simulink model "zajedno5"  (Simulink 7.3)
settings: Solver=ode3  StartTime=0.0  StopTime=350  FixedStep=0.1  RelTol=1e-3
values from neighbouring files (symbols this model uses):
  alpha_r = 3.6    [test3.m]
  alpha_u = 27    [test3.m]
  alpha_v = 26    [test3.m]
  beta_r = 0    [test3.m]
  beta_rr = 2.5    [test3.m]
  beta_u = 0    [test3.m]
  beta_uu = 56    [test3.m]
  beta_v = 0    [test3.m]
  beta_vv = 47    [test3.m]
undefined symbols (not defined in the file or in its folder): Charli, Regulatori_Charli
libraries: simulink x2, fuzblock x1

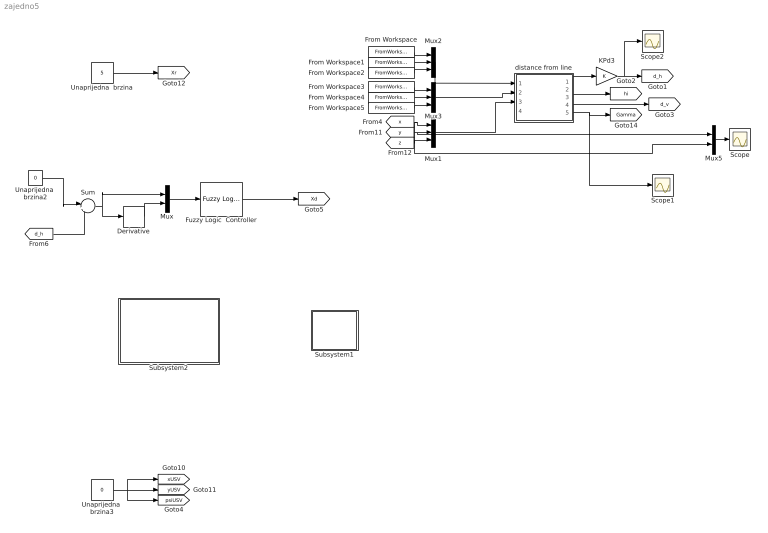
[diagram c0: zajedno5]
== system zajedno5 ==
  Derivative : Derivative
  From Workspace : FromWorkspace  VariableName=[t, n1]  SampleTime=0  Interpolate=off  OutputAfterFinalValue=Holding final value
  From Workspace1 : FromWorkspace  VariableName=[t, e1]  SampleTime=0  Interpolate=off  OutputAfterFinalValue=Holding final value
  From Workspace2 : FromWorkspace  VariableName=[t, d1]  SampleTime=0  Interpolate=off  OutputAfterFinalValue=Holding final value
  From Workspace3 : FromWorkspace  VariableName=[t, n2]  SampleTime=0  Interpolate=off  OutputAfterFinalValue=Holding final value
  From Workspace4 : FromWorkspace  VariableName=[t, e2]  SampleTime=0  Interpolate=off  OutputAfterFinalValue=Holding final value
  From Workspace5 : FromWorkspace  VariableName=[t, d2]  SampleTime=0  Interpolate=off  OutputAfterFinalValue=Holding final value
  Fuzzy Logic  Controller : fuzblock/Fuzzy Logic  Controller  SystemSampleTime=-1  fis=regulator
  KPd3 : Gain  ParameterDataType=sfix(16)  ParameterScaling=2^0  OutDataType=sfix(16)  OutScaling=2^0
  Mux : Mux  Inputs=2
  Mux1 : Mux  Inputs=3
  Mux2 : Mux  Inputs=3
  Mux3 : Mux  Inputs=3
  Mux5 : Mux  Inputs=2
  Scope : Scope
  Scope1 : Scope
  Scope2 : Scope
  Subsystem1 : Subsystem
  Subsystem2 : Subsystem
  Sum : Sum  Inputs=|+-  OutDataType=fixdt(1, 16)  OutScaling=2^0
  Unaprijedna  brzina : Constant  Value=5  OutDataType=sfix(16)  OutScaling=2^0
  Unaprijedna  brzina2 : Constant  Value=0  OutDataType=sfix(16)  OutScaling=2^0
  Unaprijedna  brzina3 : Constant  Value=0  OutDataType=sfix(16)  OutScaling=2^0
  distance from line : Subsystem
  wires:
  Mux1/1 -> distance from line/3(T0)
  [x] -> Mux1/1, Mux5/2
  [y] -> Mux1/2, Mux5/1
  [z] -> Mux1/3
  Mux2/1 -> distance from line/1(T1)
  Mux3/1 -> distance from line/2(T2)
  distance from line/1(d_h) -> KPd3/1
  distance from line/2(hi) -> [hi]
  From Workspace/1 -> Mux2/1
  From Workspace1/1 -> Mux2/2
  From Workspace2/1 -> Mux2/3
  From Workspace3/1 -> Mux3/1
  From Workspace4/1 -> Mux3/2
  From Workspace5/1 -> Mux3/3
  distance from line/4(Gamma) -> [Gamma], Scope1/1
  KPd3/1 -> [d_h], Scope2/1
  distance from line/3(d_v) -> [d_v]
  Unaprijedna  brzina2/1 -> Sum/1
  Unaprijedna  brzina3/1 -> [xUSV], [yUSV], [psiUSV]
  Mux5/1 -> Scope/1
  Sum/1 -> Mux/1, Derivative/1
  Derivative/1 -> Mux/2
  Mux/1 -> Fuzzy Logic  Controller/1
  Unaprijedna  brzina/1 -> [Xr]
  Fuzzy Logic  Controller/1 -> [Xd]
  [d_h] -> Sum/2

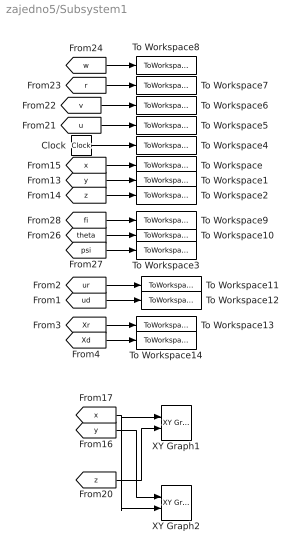
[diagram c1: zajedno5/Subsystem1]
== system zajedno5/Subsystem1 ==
  Clock : Clock
  To Workspace : ToWorkspace  VariableName=x  SampleTime=0.1  SaveFormat=Array
  To Workspace1 : ToWorkspace  VariableName=y  SampleTime=0.1  SaveFormat=Array
  To Workspace10 : ToWorkspace  VariableName=theta  SampleTime=0.1  SaveFormat=Array
  To Workspace11 : ToWorkspace  VariableName=ur  SampleTime=0.1  SaveFormat=Array
  To Workspace12 : ToWorkspace  VariableName=ud  SampleTime=0.1  SaveFormat=Array
  To Workspace13 : ToWorkspace  VariableName=Xr  SampleTime=0.1  SaveFormat=Array
  To Workspace14 : ToWorkspace  VariableName=Xd  SampleTime=0.1  SaveFormat=Array
  To Workspace2 : ToWorkspace  VariableName=z  SampleTime=0.1  SaveFormat=Array
  To Workspace3 : ToWorkspace  VariableName=psi  SampleTime=0.1  SaveFormat=Array
  To Workspace4 : ToWorkspace  VariableName=time  SampleTime=0.1  SaveFormat=Array
  To Workspace5 : ToWorkspace  VariableName=u  SampleTime=0.1  SaveFormat=Array
  To Workspace6 : ToWorkspace  VariableName=v  SampleTime=0.1  SaveFormat=Array
  To Workspace7 : ToWorkspace  VariableName=r  SampleTime=0.1  SaveFormat=Array
  To Workspace8 : ToWorkspace  VariableName=w  SampleTime=0.1  SaveFormat=Array
  To Workspace9 : ToWorkspace  VariableName=fi  SampleTime=0.1  SaveFormat=Array
  XY Graph1 : simulink/Sinks/XY Graph  SystemSampleTime=-1  xmin=-50  xmax=300  ymin=-50  ymax=300  st=-1
  XY Graph2 : simulink/Sinks/XY Graph  SystemSampleTime=-1  xmin=-5  xmax=20  ymin=-5  ymax=20  st=-1
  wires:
  [x] -> To Workspace/1
  [y] -> To Workspace1/1
  [z] -> To Workspace2/1
  Clock/1 -> To Workspace4/1
  [u] -> To Workspace5/1
  [v] -> To Workspace6/1
  [r] -> To Workspace7/1
  [w] -> To Workspace8/1
  [fi] -> To Workspace9/1
  [theta] -> To Workspace10/1
  [psi] -> To Workspace3/1
  [y] -> XY Graph2/1
  [z] -> XY Graph1/2
  [x] -> XY Graph1/1, XY Graph2/2
  [ur] -> To Workspace11/1
  [ud] -> To Workspace12/1
  [Xr] -> To Workspace13/1
  [Xd] -> To Workspace14/1

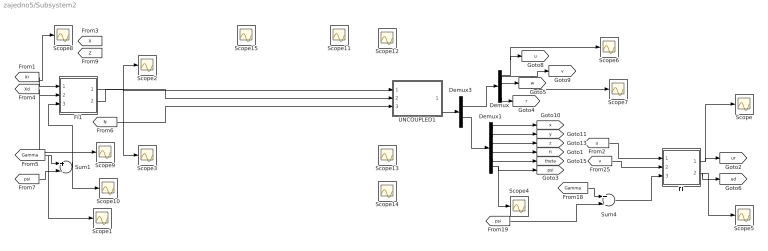
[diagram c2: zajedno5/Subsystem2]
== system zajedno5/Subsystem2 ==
  Demux : Demux  Outputs=6
  Demux1 : Demux  Outputs=6
  Demux3 : Demux  Outputs=2
  FI : Subsystem
  FI1 : Subsystem
  Scope{,1..15} (16 alike) : Scope
  Sum1 : Sum  Inputs=+-  OutDataType=sfix(16)  OutScaling=2^0
  Sum4 : Sum  Inputs=+-  OutDataType=sfix(16)  OutScaling=2^0
  UNCOUPLED1 : Subsystem  mask{u0=0, psi0=0}
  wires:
  [N] -> UNCOUPLED1/3(N)
  FI1/1(X) -> Scope2/1, UNCOUPLED1/1(X)
  FI1/2(Y) -> Scope3/1, UNCOUPLED1/2(Y)
  [Xr] -> FI1/1(Xr), Scope8/1
  [Xd] -> FI1/2(Xd), Scope9/1
  [Gamma] -> Sum1/1, Scope1/1
  Sum1/1 -> FI1/3(angle), Scope10/1
  [psi] -> Sum1/2
  Demux3/1 -> Demux/1
  Demux3/2 -> Demux1/1
  Demux/6 -> [r]
  Demux/3 -> [w]
  Demux/1 -> [u], Scope6/1
  Demux1/1 -> [x]
  Demux1/2 -> [y]
  Demux1/3 -> [z]
  Demux1/6 -> [psi], Scope4/1
  Demux/2 -> [v], Scope7/1
  UNCOUPLED1/1(Out1) -> Demux3/1
  Demux1/4 -> [fi]
  Demux1/5 -> [theta]
  [Gamma] -> Sum4/1
  Sum4/1 -> FI/3(angle)
  FI/1(ur) -> [ur], Scope/1
  FI/2(ud) -> [ud], Scope5/1
  [u] -> FI/1(u)
  [v] -> FI/2(v)
  [psi] -> Sum4/2

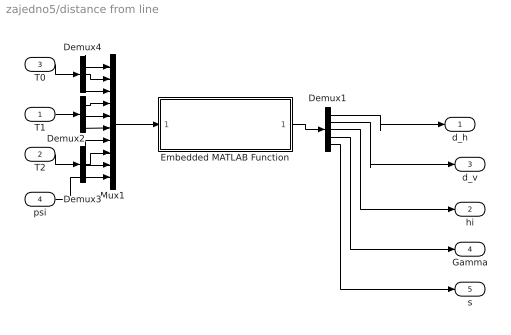
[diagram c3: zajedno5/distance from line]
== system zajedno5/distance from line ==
  T1 : Inport
  T2 : Inport  Port=2
  T0 : Inport  Port=3
  psi : Inport  Port=4
  Demux1 : Demux  Outputs=5
  Demux2 : Demux  Outputs=3
  Demux3 : Demux  Outputs=3
  Demux4 : Demux  Outputs=3
  Embedded MATLAB Function : Stateflow chart
  Mux1 : Mux  Inputs=10
  d_h : Outport  OutDataType=sfix(16)  OutScaling=2^0
  hi : Outport  Port=2  OutDataType=sfix(16)  OutScaling=2^0
  d_v : Outport  Port=3  OutDataType=sfix(16)  OutScaling=2^0
  Gamma : Outport  Port=4  OutDataType=sfix(16)  OutScaling=2^0
  s : Outport  Port=5  OutDataType=sfix(16)  OutScaling=2^0
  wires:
  Mux1/1 -> Embedded MATLAB Function/1(u)
  T1/1 -> Demux2/1
  T2/1 -> Demux3/1
  T0/1 -> Demux4/1
  Demux4/1 -> Mux1/1
  Demux4/2 -> Mux1/2
  Demux4/3 -> Mux1/3
  Demux2/1 -> Mux1/4
  Demux2/2 -> Mux1/5
  Demux2/3 -> Mux1/6
  Demux3/1 -> Mux1/7
  Demux3/2 -> Mux1/8
  Demux3/3 -> Mux1/9
  Embedded MATLAB Function/1(y) -> Demux1/1
  Demux1/1 -> d_h/1
  Demux1/2 -> d_v/1
  Demux1/3 -> hi/1
  Demux1/4 -> Gamma/1
  psi/1 -> Mux1/10
  Demux1/5 -> s/1

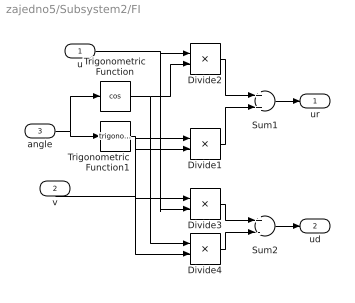
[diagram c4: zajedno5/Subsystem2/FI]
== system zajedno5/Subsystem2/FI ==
  u : Inport
  v : Inport  Port=2
  angle : Inport  Port=3
  Divide{1..4} (4 alike) : Product  Inputs=**  OutDataType=sfix(16)  OutScaling=2^-10
  Sum1 : Sum  OutDataType=sfix(16)  OutScaling=2^0
  Sum2 : Sum  Inputs=+-  OutDataType=sfix(16)  OutScaling=2^0
  Trigonometric Function : Trigonometry  Operator=cos
  Trigonometric Function1 : Trigonometry
  ur : Outport
  ud : Outport  Port=2
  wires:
  angle/1 -> Trigonometric Function1/1, Trigonometric Function/1
  Trigonometric Function/1 -> Divide4/1, Divide2/2
  u/1 -> Divide3/2, Divide2/1
  Trigonometric Function1/1 -> Divide1/1, Divide3/1
  v/1 -> Divide4/2, Divide1/2
  Divide2/1 -> Sum1/1
  Divide1/1 -> Sum1/2
  Divide3/1 -> Sum2/1
  Divide4/1 -> Sum2/2
  Sum1/1 -> ur/1
  Sum2/1 -> ud/1

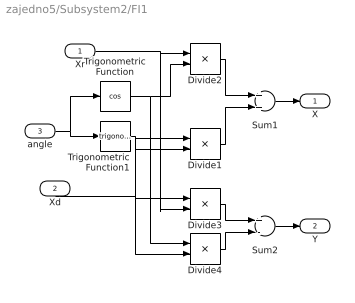
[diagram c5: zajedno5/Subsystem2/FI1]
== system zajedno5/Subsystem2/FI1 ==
  Xr : Inport
  Xd : Inport  Port=2
  angle : Inport  Port=3
  Divide{1..4} (4 alike) : Product  Inputs=**  OutDataType=sfix(16)  OutScaling=2^-10
  Sum1 : Sum  OutDataType=sfix(16)  OutScaling=2^0
  Sum2 : Sum  Inputs=+-  OutDataType=sfix(16)  OutScaling=2^0
  Trigonometric Function : Trigonometry  Operator=cos
  Trigonometric Function1 : Trigonometry
  X : Outport
  Y : Outport  Port=2
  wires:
  Sum2/1 -> Y/1
  Sum1/1 -> X/1
  Divide4/1 -> Sum2/2
  Divide3/1 -> Sum2/1
  Divide1/1 -> Sum1/2
  Divide2/1 -> Sum1/1
  Xd/1 -> Divide1/2, Divide4/2
  Trigonometric Function1/1 -> Divide3/1, Divide1/1
  Xr/1 -> Divide2/1, Divide3/2
  Trigonometric Function/1 -> Divide4/1, Divide2/2
  angle/1 -> Trigonometric Function/1, Trigonometric Function1/1

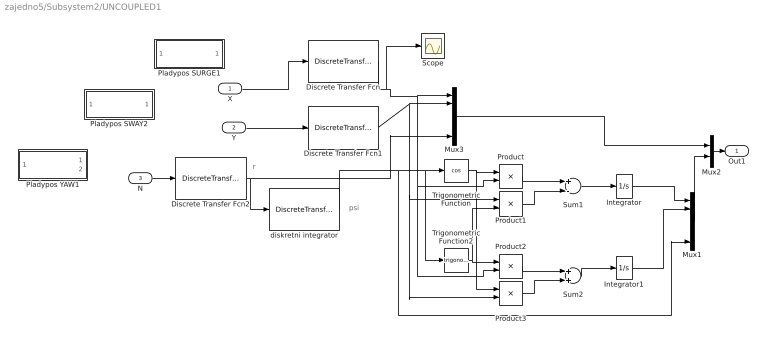
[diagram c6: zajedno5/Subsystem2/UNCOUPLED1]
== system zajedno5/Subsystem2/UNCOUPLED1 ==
  note: r
  note: psi
  X : Inport  OutDataType=fixdt(1, 16)  OutScaling=2^0
  Y : Inport  Port=2  OutDataType=fixdt(1, 16)  OutScaling=2^0
  N : Inport  Port=3  OutDataType=fixdt(1, 16)  OutScaling=2^0
  Discrete Transfer Fcn : DiscreteTransferFcn  Numerator=[0.003345]  Denominator=[1 -0.8127]  SampleTime=0.1
  Discrete Transfer Fcn1 : DiscreteTransferFcn  Numerator=[0.003519]  Denominator=[1 -0.8346]  SampleTime=0.1
  Discrete Transfer Fcn2 : DiscreteTransferFcn  Numerator=[0.02684]  Denominator=[1 -0.9329]  SampleTime=0.1
  Integrator : Integrator
  Integrator1 : Integrator
  Mux1 : Mux  Inputs=6
  Mux2 : Mux  Inputs=2
  Mux3 : Mux  Inputs=6
  Pladypos SURGE1 : Subsystem  AncestorBlock=Regulatori_Charli/Charli
  Pladypos SWAY2 : Subsystem  AncestorBlock=Regulatori_Charli/Charli
  Pladypos YAW1 : Subsystem  AncestorBlock=Regulatori_Charli/Charli
  Product{,1..3} (4 alike) : Product  OutDataType=sfix(16)  OutScaling=2^0
  Scope : Scope
  Sum1 : Sum  Inputs=+-  OutDataType=sfix(16)  OutScaling=2^0
  Sum2 : Sum  OutDataType=sfix(16)  OutScaling=2^0
  Trigonometric Function : Trigonometry  Operator=cos
  Trigonometric Function2 : Trigonometry
  diskretni integrator : DiscreteTransferFcn  Numerator=[0.1]  Denominator=[1 -1]  SampleTime=0.1
  Out1 : Outport
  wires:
  Product3/1 -> Sum2/2
  Product2/1 -> Sum2/1
  Sum2/1 -> Integrator1/1
  Sum1/1 -> Integrator/1
  Product1/1 -> Sum1/2
  Product/1 -> Sum1/1
  Integrator1/1 -> Mux1/2
  Trigonometric Function2/1 -> Product1/2, Product2/1
  Integrator/1 -> Mux1/1
  Trigonometric Function/1 -> Product3/1, Product/1
  diskretni integrator/1 -> Mux1/6, Trigonometric Function2/1, Trigonometric Function/1
  Mux1/1 -> Mux2/2
  Mux3/1 -> Mux2/1
  Mux2/1 -> Out1/1
  Discrete Transfer Fcn2/1 -> Mux3/6, diskretni integrator/1
  Discrete Transfer Fcn/1 -> Product2/2, Product/2, Mux3/1, Scope/1
  Discrete Transfer Fcn1/1 -> Product3/2, Product1/1, Mux3/2
  Y/1 -> Discrete Transfer Fcn1/1
  X/1 -> Discrete Transfer Fcn/1
  N/1 -> Discrete Transfer Fcn2/1

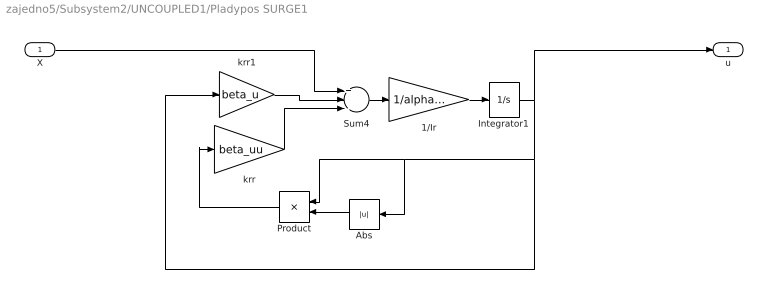
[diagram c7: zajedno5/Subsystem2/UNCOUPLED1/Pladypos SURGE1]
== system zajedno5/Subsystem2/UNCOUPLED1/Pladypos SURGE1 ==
  X : Inport  OutDataType=sfix(16)  OutScaling=2^0
  1/Ir : Gain  Gain=1/alpha_u  ParameterDataType=sfix(16)  ParameterScaling=2^0  OutDataType=sfix(16)  OutScaling=2^0
  Abs : Abs
  Integrator1 : Integrator  InitialCondition=u0  UpperSaturationLimit=30*36/225*pi/180  LowerSaturationLimit=-30*36/225*pi/180
  Product : Product  OutDataType=sfix(16)  OutScaling=2^0
  Sum4 : Sum  Inputs=+--  OutDataType=sfix(16)  OutScaling=2^0
  krr : Gain  Gain=beta_uu  ParameterDataType=sfix(16)  ParameterScaling=2^0  OutDataType=sfix(16)  OutScaling=2^0
  krr1 : Gain  Gain=beta_u  ParameterDataType=sfix(16)  ParameterScaling=2^0  OutDataType=sfix(16)  OutScaling=2^0
  u : Outport  OutDataType=sfix(16)  OutScaling=2^0
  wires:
  Integrator1/1 -> u/1, Abs/1, Product/1, krr1/1
  1/Ir/1 -> Integrator1/1
  Abs/1 -> Product/2
  Product/1 -> krr/1
  Sum4/1 -> 1/Ir/1
  krr/1 -> Sum4/3
  X/1 -> Sum4/1
  krr1/1 -> Sum4/2

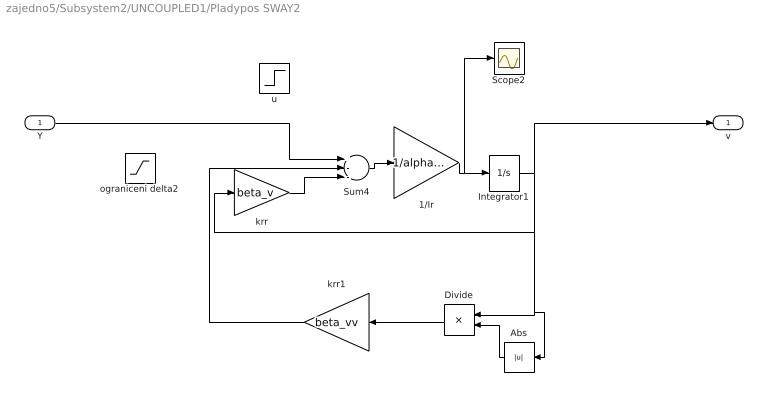
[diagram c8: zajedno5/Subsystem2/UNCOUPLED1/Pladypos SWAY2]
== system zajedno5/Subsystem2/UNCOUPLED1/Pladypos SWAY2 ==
  Y : Inport  OutDataType=sfix(16)  OutScaling=2^0
  1/Ir : Gain  Gain=1/alpha_v  ParameterDataType=sfix(16)  ParameterScaling=2^0  OutDataType=sfix(16)  OutScaling=2^0
  Abs : Abs  OutDataType=sfix(16)  OutScaling=2^0
  Divide : Product  Inputs=**  OutDataType=sfix(16)  OutScaling=2^-10
  Integrator1 : Integrator  UpperSaturationLimit=30*36/225*pi/180  LowerSaturationLimit=-30*36/225*pi/180
  Scope2 : Scope
  Sum4 : Sum  Inputs=+--  OutDataType=sfix(16)  OutScaling=2^0
  krr : Gain  Gain=beta_v  ParameterDataType=sfix(16)  ParameterScaling=2^0  OutDataType=sfix(16)  OutScaling=2^0
  krr1 : Gain  Gain=beta_vv  ParameterDataType=sfix(16)  ParameterScaling=2^0  OutDataType=sfix(16)  OutScaling=2^0
  ograniceni delta2 : Saturate  UpperLimit=1  LowerLimit=-1
  u : Step  Time=0  After=-1  SampleTime=0
  v : Outport  OutDataType=sfix(16)  OutScaling=2^0
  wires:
  Divide/1 -> krr1/1
  Abs/1 -> Divide/2
  krr/1 -> Sum4/3
  Integrator1/1 -> Abs/1, Divide/1, krr/1, v/1
  1/Ir/1 -> Integrator1/1, Scope2/1
  Sum4/1 -> 1/Ir/1
  Y/1 -> Sum4/1
  krr1/1 -> Sum4/2

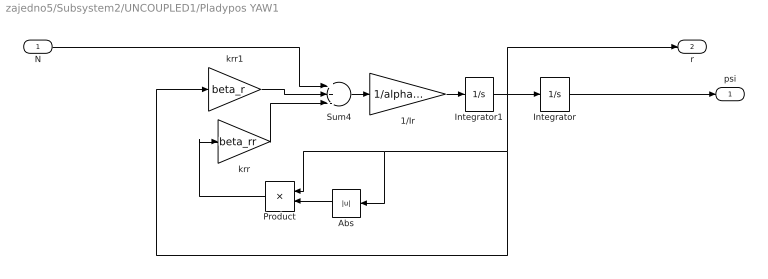
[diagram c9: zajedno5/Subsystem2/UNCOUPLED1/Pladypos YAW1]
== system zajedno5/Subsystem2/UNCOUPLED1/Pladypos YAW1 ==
  N : Inport  OutDataType=sfix(16)  OutScaling=2^0
  1/Ir : Gain  Gain=1/alpha_r  ParameterDataType=sfix(16)  ParameterScaling=2^0  OutDataType=sfix(16)  OutScaling=2^0
  Abs : Abs
  Integrator : Integrator  InitialCondition=psi0  UpperSaturationLimit=30*36/225*pi/180  LowerSaturationLimit=-30*36/225*pi/180
  Integrator1 : Integrator  UpperSaturationLimit=30*36/225*pi/180  LowerSaturationLimit=-30*36/225*pi/180
  Product : Product  OutDataType=sfix(16)  OutScaling=2^0
  Sum4 : Sum  Inputs=++-  OutDataType=sfix(16)  OutScaling=2^0
  krr : Gain  Gain=beta_rr  ParameterDataType=sfix(16)  ParameterScaling=2^0  OutDataType=sfix(16)  OutScaling=2^0
  krr1 : Gain  Gain=beta_r  ParameterDataType=sfix(16)  ParameterScaling=2^0  OutDataType=sfix(16)  OutScaling=2^0
  psi : Outport  OutDataType=sfix(16)  OutScaling=2^0
  r : Outport  Port=2  OutDataType=sfix(16)  OutScaling=2^0
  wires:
  Integrator/1 -> psi/1
  Integrator1/1 -> r/1, Integrator/1, Abs/1, Product/1, krr1/1
  1/Ir/1 -> Integrator1/1
  Abs/1 -> Product/2
  Product/1 -> krr/1
  Sum4/1 -> 1/Ir/1
  krr/1 -> Sum4/3
  N/1 -> Sum4/1
  krr1/1 -> Sum4/2

== matlab function distance from line/Embedded
MATLAB Function ==
function y = calculate_d(u)
% This block supports the Embedded MATLAB subset.
% See the help menu for details. 
x0=u(1); y0=u(2); z0=u(3);
x1=u(4); y1=u(5); z1=u(6);
x2=u(7); y2=u(8); z2=u(9);
psi=u(10);

d_h = ((x2-x1)*(y1-y0) - (x1-x0)*(y2-y1))/sqrt((x2-x1)^2+(y2-y1)^2);
Gamma = atan2(y2-y1, x2-x1);

nazivnik=sqrt((x2-x1)^2+(y2-y1)^2)*sqrt((x2-x1)^2+(y2-y1)^2+(z2-z1)^2);
d_v=(-(z2-z1)*((x0-x1)*(x2-x1)+(y0-y1)*(y2-y1))-(z1-z0)*((x2-x1)^2+(y2-y1)^2))/nazivnik;
hi=atan((z2-z1)/(sqrt((x2-x1)^2+(y2-y1)^2)));

s = cos(Gamma)*(y0 - y2) + sin(Gamma)*(x0 - x2);

y=[d_h d_v hi Gamma s];
